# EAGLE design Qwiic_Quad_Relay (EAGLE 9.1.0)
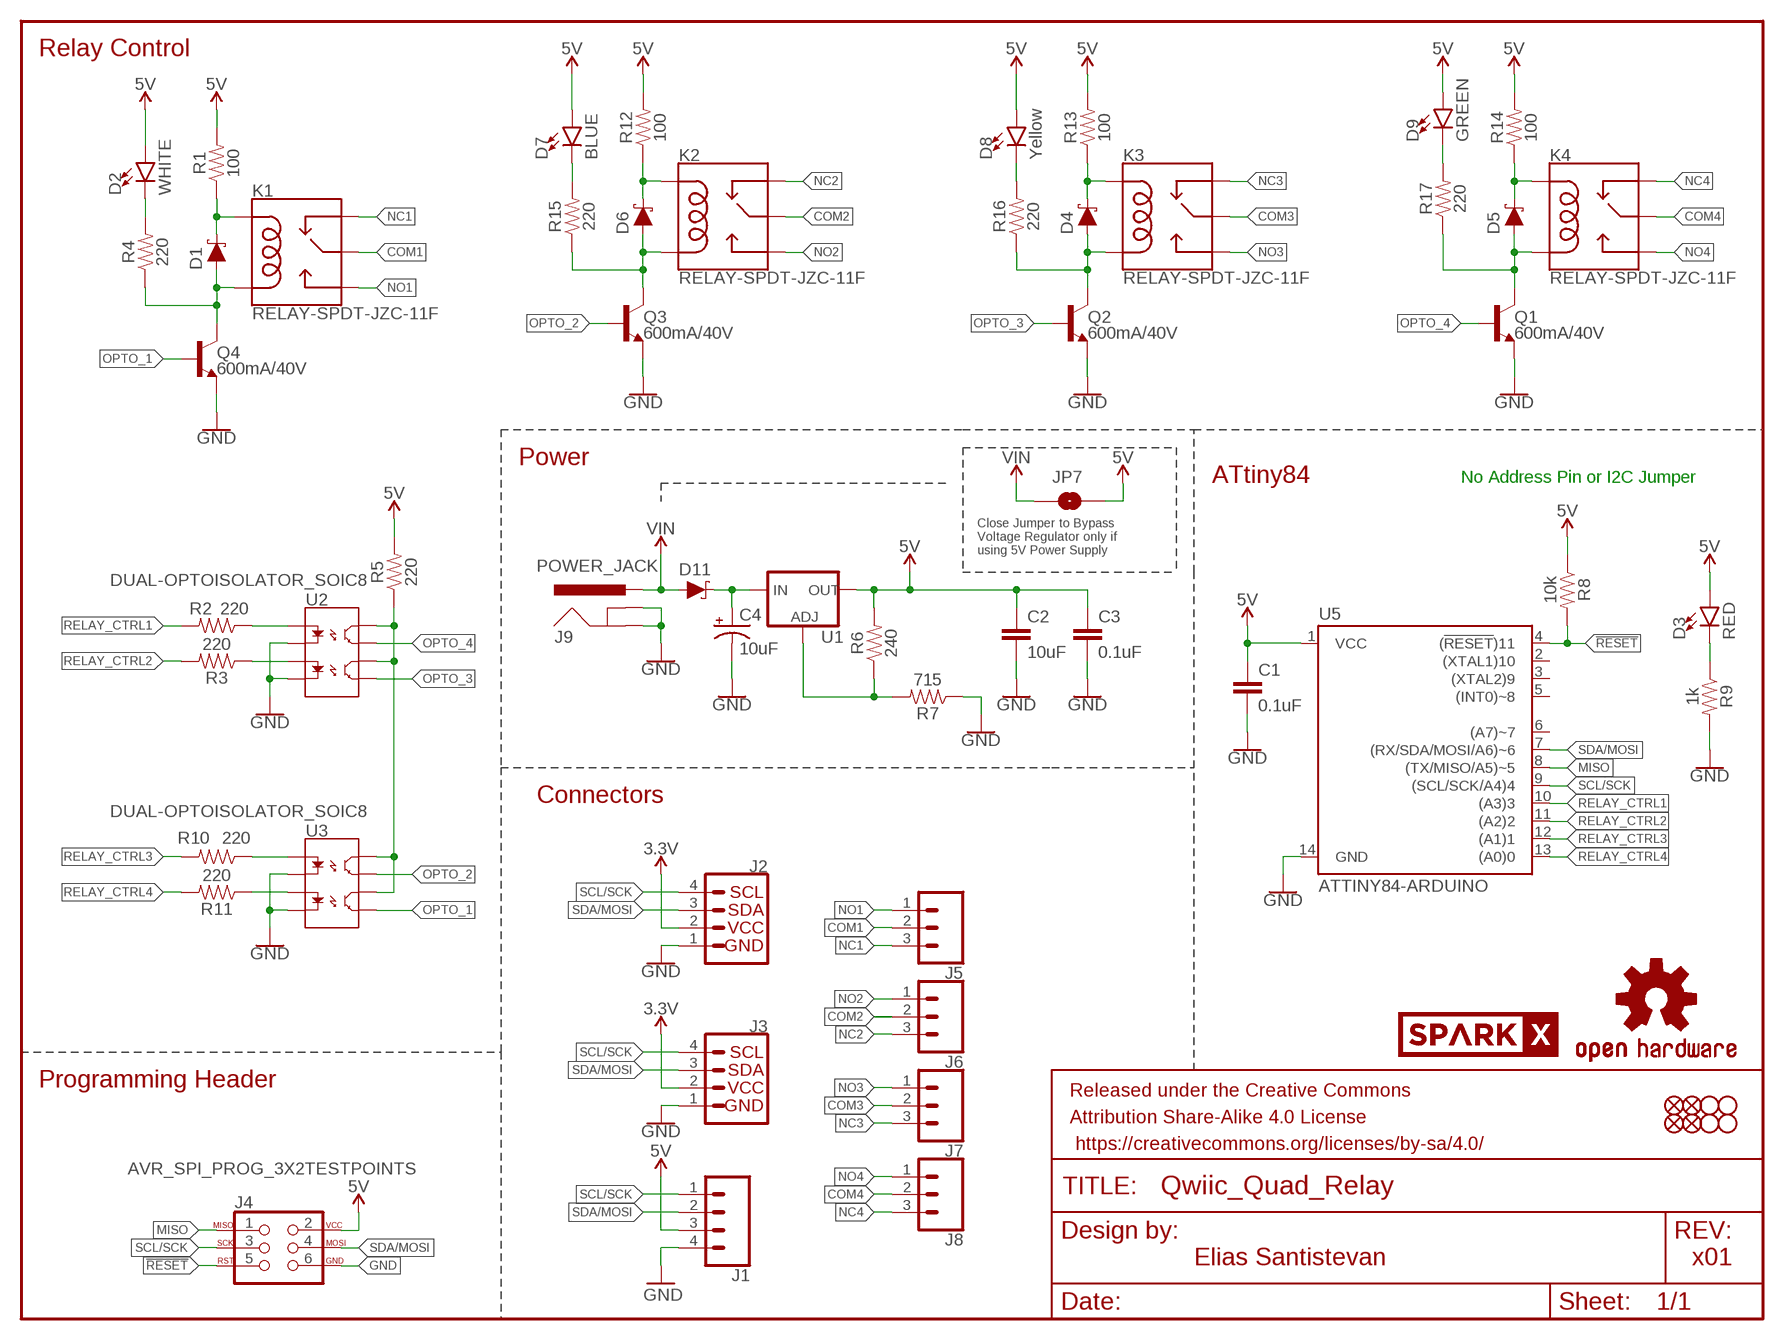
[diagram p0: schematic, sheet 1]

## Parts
C1  0.1uF  0.1UF-0603-25V-(+80/-20%)  [0603]
C2  10uF  10UF-0603-6.3V-20%  [0603]
C3  0.1uF  0.1UF-0603-25V-(+80/-20%)  [0603]
C4  10uF  10UF-POLAR-EIA3528-20V-10%(TANT)  [EIA3528]
D1  1A/23V/620mV  DIODE-SCHOTTKY-BAT20J  [SOD-323]
D2  WHITE  LED-WHITE0603  [LED-0603]
D3  RED  LED-RED0603  [LED-0603]
D4  1A/23V/620mV  DIODE-SCHOTTKY-BAT20J  [SOD-323]
D5  1A/23V/620mV  DIODE-SCHOTTKY-BAT20J  [SOD-323]
D6  1A/23V/620mV  DIODE-SCHOTTKY-BAT20J  [SOD-323]
D7  BLUE  LED-BLUE0603  [LED-0603]
D8  Yellow  LED-YELLOW0603  [LED-0603]
D9  GREEN  LED-GREEN0603  [LED-0603]
D11  1A/40V/500mV  DIODE-SCHOTTKY-SS14  [SMA-DIODE]
FRAME1  FRAME-LETTER  [CREATIVE_COMMONS]
J1  CONN_041X04_NO_SILK  [1X04_NO_SILK]
J2  Qwiic Right Angle  I2C_STANDARDQWIIC  [1X04_1MM_RA]
J3  Qwiic Right Angle  I2C_STANDARDQWIIC  [1X04_1MM_RA]
J4  AVR_SPI_PROG_3X2TESTPOINTS  [2X3_TEST_POINTS]
J5  CONN_03-SCREW-5MM  [SCREWTERMINAL-5MM-3]
J6  CONN_03-SCREW-5MM  [SCREWTERMINAL-5MM-3]
J7  CONN_03-SCREW-5MM  [SCREWTERMINAL-5MM-3]
J8  CONN_03-SCREW-5MM  [SCREWTERMINAL-5MM-3]
J9  POWER_JACK  [POWER_JACK_PTH]
JP1  STAND-OFF  [STAND-OFF]
JP2  FIDUCIAL1X2  [FIDUCIAL-1X2]
JP3  STAND-OFF  [STAND-OFF]
JP4  STAND-OFF  [STAND-OFF]
JP5  STAND-OFF  [STAND-OFF]
JP6  FIDUCIAL1X2  [FIDUCIAL-1X2]
JP7  JUMPER-SMT_2_NO_SILK  [SMT-JUMPER_2_NO_SILK]
JP8  FIDUCIAL1X2  [FIDUCIAL-1X2]
JP9  FIDUCIAL1X2  [FIDUCIAL-1X2]
K1  RELAY-SPDT-JZC-11F  [RELAY-JZC]
K2  RELAY-SPDT-JZC-11F  [RELAY-JZC]
K3  RELAY-SPDT-JZC-11F  [RELAY-JZC]
K4  RELAY-SPDT-JZC-11F  [RELAY-JZC]
LOGO1  OSHW-LOGOS  [OSHW-LOGO-S]
Q1  600mA/40V  TRANS_NPN-MMBT2222AL  [SOT23-3]
Q2  600mA/40V  TRANS_NPN-MMBT2222AL  [SOT23-3]
Q3  600mA/40V  TRANS_NPN-MMBT2222AL  [SOT23-3]
Q4  600mA/40V  TRANS_NPN-MMBT2222AL  [SOT23-3]
R1  100  100OHM-0603-1/10W-1%  [0603]
R2  220  220OHM-0603-1/10W-1%  [0603]
R3  220  220OHM-0603-1/10W-1%  [0603]
R4  220  220OHM-0603-1/10W-1%  [0603]
R5  220  220OHM-0603-1/10W-1%  [0603]
R6  240  240OHM-0603-1/10W-1%  [0603]
R7  715  715OHM-0603-1/10W-1%  [0603]
R8  10k  10KOHM-0603-1/10W-1%  [0603]
R9  1k  1KOHM-0603-1/10W-1%  [0603]
R10  220  220OHM-0603-1/10W-1%  [0603]
R11  220  220OHM-0603-1/10W-1%  [0603]
R12  100  100OHM-0603-1/10W-1%  [0603]
R13  100  100OHM-0603-1/10W-1%  [0603]
R14  100  100OHM-0603-1/10W-1%  [0603]
R15  220  220OHM-0603-1/10W-1%  [0603]
R16  220  220OHM-0603-1/10W-1%  [0603]
R17  220  220OHM-0603-1/10W-1%  [0603]
U1  V_REG_LM1117SOT223  [SOT223]
U2  DUAL-OPTOISOLATOR_SOIC8  [SO08]
U3  DUAL-OPTOISOLATOR_SOIC8  [SO08]
U5  ATTINY84-ARDUINO  [SO14]
U$12  SPARKX-LOGO4  [SPARKX-MEDIUM]

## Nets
3.3V: J2.2 J3.2
5V: C1.1 C2.1 C3.1 D2.A D3.A D7.A D8.A D9.A J1.3 J4.2 JP7.2 R1.2 R5.2 R6.2 R8.1 R12.2 R13.2 R14.2 U1.2(OUT) U1.4(OUT) U5.1(VCC)
!RESET: J4.5 R8.2 U5.4((!RESET!)11)
COM1: J5.2 K1.4(MAIN)
COM2: J6.2 K2.4(MAIN)
COM3: J7.2 K3.4(MAIN)
COM4: J8.2 K4.4(MAIN)
GND: C1.2 C2.2 C3.2 C4.C(-) J1.4 J2.1 J3.1 J4.6 J9.GND J9.GNDBREAK Q1.2(E) Q2.2(E) Q3.2(E) Q4.2(E) R7.1 R9.2 U2.2(C1) U2.4(C2) U3.2(C1) U3.4(C2) U5.14(GND)
MISO: J4.1 U5.8((TX/MISO/A5)~5)
N$1: D6.C K2.5(COIL1) R12.1
N$2: D1.A K1.1(COIL2) Q4.3(C) R4.1
N$3: R11.1 U3.3(A2)
N$4: C4.A(+) D11.C U1.3(IN)
N$5: R10.1 U3.1(A1)
N$6: R5.1 U2.6(CL2) U2.8(CL1) U3.6(CL2) U3.8(CL1)
N$7: D1.C K1.5(COIL1) R1.1
N$8: D2.C R4.2
N$9: R2.1 U2.1(A1)
N$11: R3.1 U2.3(A2)
N$12: D6.A K2.1(COIL2) Q3.3(C) R15.1
N$13: D3.C R9.1
N$14: D4.C K3.5(COIL1) R13.1
N$15: D4.A K3.1(COIL2) Q2.3(C) R16.1
N$16: D5.C K4.5(COIL1) R14.1
N$17: D5.A K4.1(COIL2) Q1.3(C) R17.1
N$19: R6.1 R7.2 U1.1(ADJ)
N$20: D9.C R17.2
N$21: D8.C R16.2
N$22: D7.C R15.2
NC1: J5.3 K1.2(NC)
NC2: J6.3 K2.2(NC)
NC3: J7.3 K3.2(NC)
NC4: J8.3 K4.2(NC)
NO1: J5.1 K1.3(NO)
NO2: J6.1 K2.3(NO)
NO3: J7.1 K3.3(NO)
NO4: J8.1 K4.3(NO)
OPTO_1: Q4.1(B) U3.5(EM2)
OPTO_2: Q3.1(B) U3.7(EM1)
OPTO_3: Q2.1(B) U2.5(EM2)
OPTO_4: Q1.1(B) U2.7(EM1)
RELAY_CTRL1: R2.2 U5.10((A3)3)
RELAY_CTRL2: R3.2 U5.11((A2)2)
RELAY_CTRL3: R10.2 U5.12((A1)1)
RELAY_CTRL4: R11.2 U5.13((A0)0)
SCL/SCK: J1.1 J2.4 J3.4 J4.3 U5.9((SCL/SCK/A4)4)
SDA/MOSI: J1.2 J2.3 J3.3 J4.4 U5.7((RX/SDA/MOSI/A6)~6)
VIN: D11.A J9.PWR JP7.1
Unconnected: U5.2((XTAL1)10) U5.3((XTAL2)9) U5.5((INT0)~8) U5.6((A7)~7)

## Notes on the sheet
- Relay Control
- Power
- ATtiny84 | No Address Pin or I2C Jumper
- Close Jumper to Bypass
  Voltage Regulator only if 
  using 5V Power Supply
- Connectors
- Programming Header
- Elias Santistevan | x01

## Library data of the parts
C1 C3 = SparkFun-Capacitors:0.1UF: 0.1µF ceramic capacitors; PROD_ID: CAP-00810
C2 = SparkFun-Capacitors:10UF: 10.0µF ceramic capacitors; PROD_ID: CAP-11015
C4 = SparkFun-Capacitors:10UF-POLAR: 10.0µF polarized capacitors; PROD_ID: CAP-08063
D1 D4-D6 = SparkFun-DiscreteSemi:DIODE-SCHOTTKY: Schottky diode; PROD_ID: DIO-11623
D2 = SparkFun-LED:LED-WHITE: White SMD LED; PROD_ID: DIO-09004
D3 = SparkFun-LED:LED-RED: Red SMD LED; PROD_ID: DIO-00819
D7 = SparkFun-LED:LED-BLUE: Blue SMD LED; PROD_ID: DIO-08575
D8 = SparkFun-LED:LED-YELLOW: Yellow SMD LED; PROD_ID: DIO-09003
D9 = SparkFun-LED:LED-GREEN: Green SMD LED; PROD_ID: DIO-00821
D11 = SparkFun-DiscreteSemi:DIODE-SCHOTTKY: Schottky diode; PROD_ID: DIO-08053
FRAME1 = SparkFun-Aesthetics:FRAME-LETTER: Schematic Frame - Letter
J1 = SparkFun-Connectors:CONN_04: Multi connection point. Often used as Generic Header-pin footprint for 0.1 inch spaced/style header connections On any of the 0.1 inch spaced packages, you can populate with these: Break Away Headers - Straight (PRT-00116) Break Away Male Headers - Right Angle (PRT-00553) Female Headers (PRT-00115)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; PROD_ID: CONN-09696
J2 J3 = SparkFun-Connectors:I2C_STANDARD: SparkFun I2C Standard Pinout Header SparkFun has standardized on a pinout for all I2C based sensor breakouts. This pinout allows I2C boards to be plugged directly into the headers on Arduino Uno compatible boards, and to be daisy chained easily. Example SparkFun Products: SparkFun Atmospheric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; PROD_ID: CONN-13694
J4 = SparkFun-Connectors:AVR_SPI_PROG_3X2: AVR ISP 6 Pin This is the reduced ISP connector for AVR programming. Common on Arduino. This footprint will take up less PCB space and can be used with a 10-pin to 6-pin adapter such as SKU: BOB-08508 **Special note about "TEST_POINT" package. The stop mask is on the top side, so if you want your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
J5-J8 = SparkFun-Connectors:CONN_03: Multi connection point. Often used as Generic Header-pin footprint for 0.1 inch spaced/style header connections On any of the 0.1 inch spaced packages, you can populate with these: Break Away Headers - Straight (PRT-00116) Break Away Male Headers - Right Angle (PRT-00553) Female Headers (PRT-00115)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; PROD_ID: CONN-10134; SF_SKU: PRT-08433
J9 = SparkFun-Connectors:POWER_JACK: Power Jack Connector This is the standard 5.5mm barrel jack for power. The PTH is the most common, proven, reliable, footprint. The Slot footprint only works if the mill layer is transmitted to the PCB fab house so be warned. Here are the connectors we sell at SparkFun: DC Barrel Power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; PROD_ID: CONN-08197
JP1 JP3-JP5 = SparkFun:STAND-OFF: Stand Off
JP2 JP6 JP8 JP9 = SparkFun-Aesthetics:FIDUCIAL: Fiducial Alignment Points
JP7 = SparkFun-Jumpers:JUMPER-SMT_2_NO: Normally open jumper
K1-K4 = SparkFun-Electromechanical:RELAY-SPDT: SPDT Electromechanical Relay Single-pole, double-throw sealed relays. When current is applied to the coil, it throws a simple changeover switch, terminating the connection from the NC contact to ground and closing the NO contact. Use them to switch high voltage/high current devices. SparkFun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; PROD_ID: COMP-09533; SF_SKU: COM-00100
LOGO1 = SparkFun-Aesthetics:OSHW-LOGO: Open-Source Hardware (OSHW) Logo
Q1-Q4 = SparkFun-DiscreteSemi:TRANS_NPN: NPN transistor Current controlled devices typically used to amplify current or used as a switch. BC547 - COM-08928 (TO-92 45V 100mA) (1.Collector 2.Base 3.Emitter) 2N3904 - COM-00521 (TO-92 40V 200mA) (1.Emitter 2.Base 3.Collector) P2N2222A - COM-12852 (TO-92 40V 600mA) (1.Collector 2.Base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; PROD_ID: TRANS-08049
R1 R12-R14 = SparkFun-Resistors:100OHM: 100Ω resistor; PROD_ID: RES-07863
R2-R5 R10 R11 R15-R17 = SparkFun-Resistors:220OHM: 220Ω resistor; PROD_ID: RES-07861
R6 = SparkFun-Resistors:240OHM: 240Ω resistor; PROD_ID: RES-07849
R7 = SparkFun-Resistors:715OHM: 715Ω resistor; PROD_ID: RES-07850
R8 = SparkFun-Resistors:10KOHM: 10kΩ resistor; PROD_ID: RES-00824
R9 = SparkFun-Resistors:1KOHM: 1kΩ resistor; PROD_ID: RES-07856
U1 = SparkFun-IC-Power:V_REG_LM1117: Voltage Regulator LM1117 Standard adjustable voltage regulator but in SMD form. Spark Fun Electronics SKU : COM-00595; PROD_ID: VREG-08170
U2 U3 = SparkFun-DiscreteSemi:DUAL-OPTOISOLATOR: Optocoupler, Phototransistor Output, Dual Channel Optically coupled pairs with a gallium arsenide infrared LED and a silicon NPN phototransistor. Signal information, including a DC level, can be transmitted by the device while maintaining a high degree of electrical isolation between input and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; PROD_ID: IC-09076
U5 = SparkFun-IC-Microcontroller:ATTINY84-ARDUINO; PROD_ID: IC-11285
U$12 = SparkX:SPARKX-LOGO

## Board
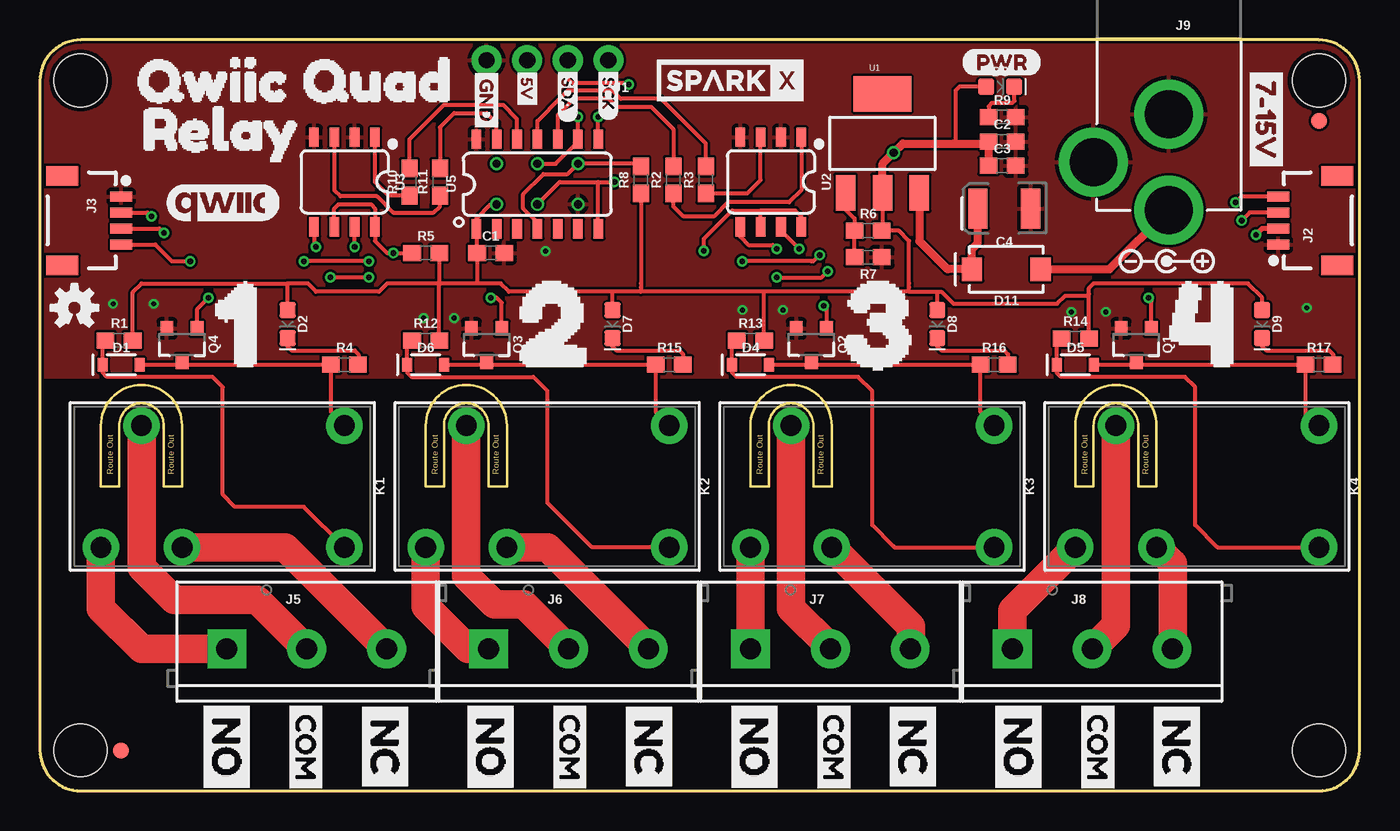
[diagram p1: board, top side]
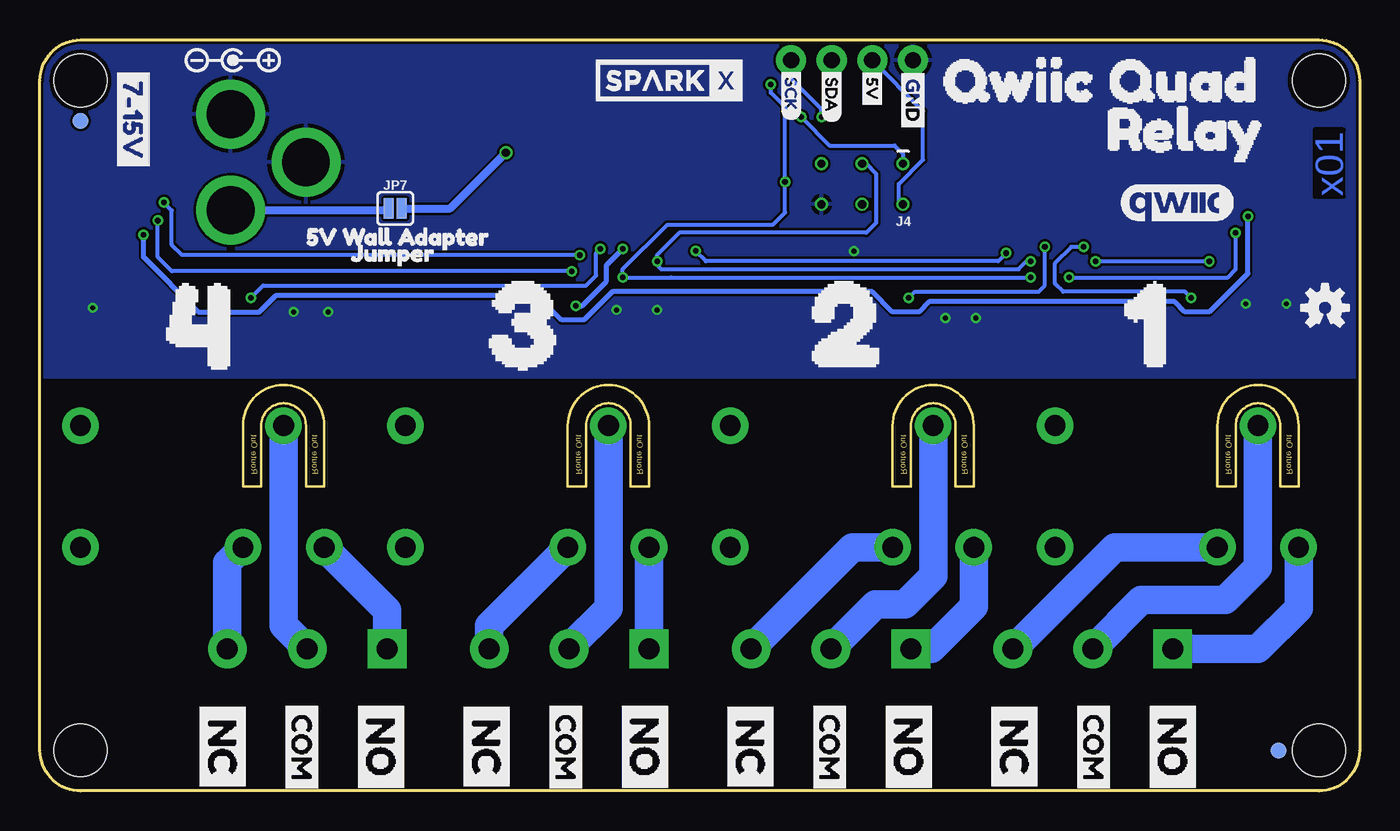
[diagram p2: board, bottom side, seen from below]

Size 82.55 x 46.99 mm. Coordinates in mm from the lower left corner, seen from the top.
Outline: 80.01,46.99 2.54,46.99 arc90 0,44.45 0,2.54 arc90 2.54,0 80.01,0 arc90 82.55,2.54 82.55,44.45 arc90 80.01,46.99
Copper layers (1*16): Top 0.035mm / dielectric 1.5mm / Bottom 0.035mm
Design rules "SparkFun-2-layer-PCBWay-LIMIT": minimum track width 6mil, minimum drill 0.3mm, track to track 6mil, track to pad 6mil, pad to pad 6mil, via to via 6mil, smd to smd 6mil, copper to edge 6mil, drill to drill 6mil, minimum pad ring 6mil, minimum via ring 6mil, stop-mask expansion 4mil, vias tented up to drill 25mil, thermal gap 10mil
Milling: 40 lines

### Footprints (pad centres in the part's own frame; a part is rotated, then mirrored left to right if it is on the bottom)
0603 = smd 1.1 x 1: 1 -0.85,0; 2 0.85,0
EIA3528 = smd 1.2 x 2.5: A 1.65,0; C -1.65,0
SOD-323 = smd 0.63 x 0.83: A 1.15,0; C -1.15,0
LED-0603 = smd 1 x 1: A -0.877,0; C 0.877,0
SMA-DIODE = smd 1.27 x 1.47: A -2.15,0; C 2.15,0
1X04_NO_SILK = drill 1.016 pad 1.88: 1 0,0; 2 2.54,0; 3 5.08,0; 4 7.62,0
1X04_1MM_RA = smd 0.6 x 1.35: 1 -1.5,0; 2 -0.5,0; 3 0.5,0; 4 1.5,0 | smd 1.2 x 2: NC1 2.8,-3.675; NC2 -2.8,-3.675
2X3_TEST_POINTS = drill 0.508: 1 -2.54,-1.27; 2 -2.54,1.27; 3 0,-1.27; 4 0,1.27; 5 2.54,-1.27; 6 2.54,1.27
SCREWTERMINAL-5MM-3 = drill 1.3 pad 2.413 square: 1 0,0 | drill 1.3 pad 2.413: 2 5,0; 3 10,0
POWER_JACK_PTH = drill 2.997 pad 4.318: GND 0,7.7; GNDBREAK 4.7,10.7; PWR 0,13.7
STAND-OFF = hole 3.302: 0,0
FIDUCIAL-1X2 = smd 1 x 1: 1 0,0
SMT-JUMPER_2_NO_SILK = smd 0.635 x 1.27: 1 -0.406,0; 2 0.406,0
RELAY-JZC = drill 1.3 pad 2.286: 1 3.81,-8.89; 2 -3.81,1.27; 3 -3.81,6.35; 4 3.81,3.81; 5 -3.81,-8.89
SOT23-3 = smd 0.8 x 0.9: 1 -0.95,-1; 2 0.95,-1; 3 0,1.1
SOT223 = smd 1.219 x 2.235: 1 -2.311,-3.099; 2 0,-3.099; 3 2.311,-3.099 | smd 3.6 x 2.2: 4 0,3.099
SO08 = smd 0.6 x 1.2: 1 -1.905,-2.8; 2 -0.635,-2.8; 3 0.635,-2.8; 4 1.905,-2.8; 5 1.905,2.8; 6 0.635,2.8; 7 -0.635,2.8; 8 -1.905,2.8
SO14 = smd 0.6 x 1.2: 1 -3.175,-2.8; 2 -1.905,-2.8; 3 -0.635,-2.8; 4 0.635,-2.8; 5 1.905,-2.8; 6 3.175,-2.8; 7 4.445,-2.8; 8 4.445,2.8; 9 3.175,2.8; 10 1.905,2.8; 11 0.635,2.8; 12 -0.635,2.8; 13 -1.905,2.8; 14 -3.175,2.8

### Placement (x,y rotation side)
C1  28.19,33.66 0 top
C2  60.2,40.64 0 top
C3  60.2,39.12 0 top
C4  60.33,36.45 180 top
D1  5.08,26.67 0 top
D2  15.49,29.21 270 top
D3  60.07,44.07 0 top
D4  44.45,26.67 0 top
D5  64.77,26.67 0 top
D6  24.13,26.67 0 top
D7  35.81,29.21 270 top
D8  56.13,29.21 270 top
D9  76.45,29.21 270 top
D11  60.45,32.64 180 top
FRAME1  not placed on the board
J1  35.56,45.72 180 top
J2  77.47,35.69 90 top
J3  5.08,35.69 270 top
J4  31.11,37.97 180 bottom
J5  11.68,8.89 0 top
J6  28.07,8.89 0 top
J7  44.45,8.89 0 top
J8  60.83,8.89 0 top
J9  70.61,50.04 180 top
JP1  2.54,2.54 0 top
JP2  80.01,41.91 0 bottom
JP3  2.54,44.45 0 top
JP4  80.01,44.45 0 top
JP5  80.01,2.54 0 top
JP6  5.08,2.54 0 bottom
JP7  60.33,36.45 0 bottom
JP8  5.08,2.54 0 top
JP9  80.01,41.91 0 top
K1  10.16,19.05 90 top
K2  30.48,19.05 90 top
K3  50.8,19.05 90 top
K4  71.12,19.05 90 top
LOGO1  2.16,30.23 0 top
Q1  68.58,27.94 180 top
Q2  48.26,27.94 180 top
Q3  27.94,27.94 180 top
Q4  8.89,27.94 180 top
R1  4.95,28.19 0 top
R2  39.62,38.23 90 top
R3  41.66,38.23 90 top
R4  19.05,26.67 0 top
R5  24.13,33.66 0 top
R6  51.82,35.05 0 top
R7  51.82,33.4 180 top
R8  37.59,38.23 90 top
R9  60.2,42.16 0 top
R10  23.11,38.1 90 top
R11  25.02,38.1 90 top
R12  24.13,28.19 0 top
R13  44.45,28.19 0 top
R14  64.77,28.32 0 top
R15  39.37,26.67 0 top
R16  59.69,26.67 0 top
R17  80.01,26.67 0 top
U1  52.7,40.51 0 top
U2  45.72,38.1 180 top
U3  19.05,38.1 180 top
U5  30.48,37.97 0 top
U$1  [PWR-()-04]  57.66,45.59 0 top
U$2  [20]  25.4,29.21 0 top
U$3  [10]  6.35,29.21 0 top
U$4  [30]  45.72,29.21 0 top
U$5  [40]  66.04,29.21 0 top
U$6  [QWIIC_QUAD_0]  3.81,44.45 0 top
U$7  [RELAY0]  4.19,41.4 0 top
U$8  [SCK-[)-03]  35.56,45.34 270 top
U$9  [GND-03]  27.94,45.34 270 top
U$10  [5V0]  30.48,45.34 270 top
U$11  [SDA0]  33.02,45.34 270 top
U$12  43.18,44.45 0 top
U$13  [OSHW-LOGO-S]  2.16,30.23 0 bottom
U$14  [SPARKX-MEDIUM]  43.18,44.45 0 bottom
U$15  [NO0]  11.68,6.22 270 top
U$16  [COM0]  16.64,5.97 270 top
U$17  [NC0]  21.59,6.1 270 top
U$18  [NO0]  28.19,6.22 270 top
U$19  [COM0]  33.15,5.97 270 top
U$20  [NC0]  38.1,6.1 270 top
U$21  [NO0]  44.7,6.22 270 top
U$22  [COM0]  49.66,5.97 270 top
U$23  [NC0]  54.61,6.1 270 top
U$24  [NO0]  61.21,6.22 270 top
U$25  [COM0]  66.17,5.97 270 top
U$26  [NC0]  71.12,6.1 270 top
U$27  [NO0]  44.7,6.22 270 bottom
U$28  [COM0]  66.17,5.97 270 bottom
U$29  [NC0]  71.12,6.1 270 bottom
U$30  [NO0]  61.21,6.22 270 bottom
U$31  [COM0]  49.66,5.97 270 bottom
U$32  [NC0]  54.61,6.1 270 bottom
U$33  [NO0]  28.19,6.22 270 bottom
U$34  [COM0]  33.15,5.97 270 bottom
U$35  [NC0]  38.1,6.1 270 bottom
U$36  [NO0]  11.68,6.22 270 bottom
U$37  [COM0]  16.64,5.97 270 bottom
U$38  [NC0]  21.59,6.1 270 bottom
U$39  [10]  19.3,29.21 0 bottom
U$40  [20]  38.86,29.21 0 bottom
U$41  [30]  59.05,29.21 0 bottom
U$42  [40]  79.25,29.08 0 bottom
U$43  [QWIIC_QUAD_0]  28.32,44.45 0 bottom
U$44  [RELAY0]  18.03,41.4 0 bottom
U$45  [GND-03]  27.94,45.34 270 bottom
U$46  [5V0]  30.48,45.34 270 bottom
U$47  [SDA0]  33.02,45.34 270 bottom
U$48  [SCK-[)-03]  35.56,45.34 270 bottom
U$49  [7#15V0]  76.71,45.59 270 top
U$50  [5V_WALL_ADAPTER0]  66.8,34.67 0 bottom
U$51  [POLARITY_MARKING_CENTER_POSITIVE#JPG]  70.48,33.15 0 top
U$52  [JUMPER0]  64.01,33.66 0 bottom
U$53  [7#15V0]  76.71,45.59 270 bottom
U$54  [POLARITY_MARKING_CENTER_POSITIVE#JPG]  70.48,45.72 0 bottom
U$55  [QWIIC#JPG]  11.43,36.83 0 top
U$57  [QWIIC#JPG]  11.43,36.83 0 bottom

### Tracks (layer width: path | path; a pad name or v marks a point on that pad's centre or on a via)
3.3V  (via drill 0.35)
  Top 0.254: J3.2 6.74,36.19 v6.99,35.94
  Top 0.305: J2.2 76.46,35.19 v76.07,34.8
  Bottom 0.305: v6.99,35.94 6.99,32.38 9.4,29.97 10.92,29.97 11.56,30.61 26.92,30.61 27.56,29.97 29.21,29.97 30.48,31.24 46.74,31.24 48.51,29.46 49.91,29.46 51.44,30.99 67.82,30.99 68.83,29.97 72.64,29.97 76.07,33.4 v76.07,34.8
5V  (via drill 0.51)
  Top 0.254: 54.37,31.24 45.3,31.24 | 45.3,31.24 37.59,31.24 | R8.1 37.59,31.75 37.59,31.5 37.59,31.24 | 15.49,31.75 6.35,31.75 5.8,31.2 R1.2 | D9.A 76.45,30.86 75.56,31.75 65.91,31.75 65.66,31.5 65.62,31.46 65.62,31.11 | D2.A 15.49,31.75 | J4.2 28.19,36.7 27.3,35.81 U5.1 27.34,35.13 C1.1 27.34,31.79 27.3,31.75 | D3.A 57.53,44.07 57.28,43.81 57.28,40.64 57.15,40.51 | U1.2 52.7,35.09 | 52.7,35.09 R6.2 | 52.7,35.09 52.74,35.05 53.72,35.05 54.37,34.41 54.37,31.75 54.37,31.5 54.37,31.24 | R14.2 65.62,31.11 | R13.2 45.3,31.24 | 37.59,31.24 35.81,31.24 | 35.81,31.24 29.34,31.24 28.83,31.75 27.3,31.75 | 27.3,31.75 25.02,31.75 | 25.02,31.75 24.89,31.75 | 24.89,31.75 21.72,31.75 21.21,31.24 17.27,31.24 16.76,31.75 15.49,31.75 | R12.2 24.98,31.66 24.89,31.75 | 25.02,31.75 24.98,31.79 R5.2 | D7.A 35.81,31.24 | 54.37,31.24 56.13,31.24 | 56.13,31.24 56.39,31.24 57.15,30.48 63.63,30.48 64.14,30.99 65.49,30.99 65.62,31.11 | D8.A 56.13,31.24
  Top 0.508: C3.1 C2.1 59.22,40.51 57.15,40.51 53.98,40.51 v53.4,39.94 52.7,39.24 U1.2
  Bottom 0.254: J1.3 27.3,42.55 27.3,39.5 28.83,37.97 28.83,36.96 J4.2
  Bottom 0.508: JP7.2 56.9,36.45 v53.4,39.94
!RESET
  Top 0.254: U5.4 31.11,35.55 30.23,36.44 30.23,37.34 31.5,38.61 33.02,38.61 J4.5 37.43,39.24 R8.2
COM1
  Top 1.778: K1.4 6.35,13.97 8.38,11.94 8.89,11.94 13.59,11.94 16.64,8.89 J5.2
  Bottom 1.778: K1.4 6.35,13.97 8.38,11.94 13.64,11.94 J5.2
COM2
  Top 1.778: K2.4 26.67,13.46 28.45,11.68 30.27,11.68 J6.2
  Bottom 1.778: K2.4 26.67,13.46 28.45,11.68 30.27,11.68 J6.2 | J6.2
COM3
  Top 1.778: K3.4 46.99,11.43 49.45,8.97 J7.2
  Bottom 1.778: K3.4 46.99,11.43 49.45,8.97 J7.2
COM4
  Top 1.778: K4.4 67.31,10.37 J8.2 | K4.4
  Bottom 1.778: K4.4 67.31,10.37 J8.2 | K4.4
GND  (via drill 0.3)
  other vias: 46.48,30.1 66.67,29.97 25.91,29.59 7.11,30.48 64.52,29.97 79.25,30.23 43.94,30.1 4.57,30.48 24,29.59 31.62,33.78
  pour Bottom: 0,25.91 82.55,25.91 82.55,46.99 0,46.99
  pour Top: 0,25.91 0,46.99 82.55,46.99 82.55,25.91
MISO  (via drill 0.35)
  Top 0.254: U5.8 v34.92,42.16
  Bottom 0.254: v34.92,42.16 33.15,40.39 29.08,40.39 28.57,39.88 J4.1
N$1
  Top 0.254: K2.5 34.54,15.24 31.75,18.03 31.75,25.02 30.99,25.78 30.86,25.91 23.24,25.91 22.98,26.17 D6.C 22.98,27.89 R12.1
N$2
  Top 0.254: D1.A 8.72,26.67 Q4.3 9.06,26.67 R4.1 18.2,23.71 K1.1
N$3
  Top 0.254: U3.3 18.41,37.59 18.8,37.21 21.08,37.21 22.1,36.2 24.64,36.2 25.02,36.58 R11.1
N$4
  Top 0.508: U1.3 55.02,34.39 56.13,33.27 56.77,32.64 D11.C 58.3,33.92 58.67,34.29 C4.A
N$5
  Top 0.254: R10.1 21.8,37.25 20.95,38.1 U3.1
N$6  (via drill 0.35)
  Top 0.254: U3.6 18.41,36.45 18.67,36.7 20.7,36.7 20.95,36.45 U3.8 20.95,34.42 21.72,33.66 v22.1,33.66 R5.1 | 45.09,36.32 46.99,36.32 47.24,36.32 47.62,35.94 U2.8 | U2.6 45.09,36.32 | v41.53,33.78 41.53,34.54 43.31,36.32 45.09,36.32
  Bottom 0.254: v41.53,33.78 40.89,33.15 22.61,33.15 v22.1,33.66
N$7
  Top 0.254: R1.1 3.93,28.02 D1.C 3.93,26.17 4.19,25.91 10.79,25.91 11.43,25.27 11.43,18.54 12.19,17.78 16.51,17.78 K1.5
N$8
  Top 0.254: R4.2 19.93,26.7 19.93,27.32 19.68,27.56 15.75,27.56 15.49,27.81 D2.C
N$9
  Top 0.254: U2.1 47.62,37.59 46.86,36.83 43.05,36.83 42.16,35.94 40.26,35.94 39.62,36.58 R2.1
N$11
  Top 0.254: U2.3 45.09,38.23 44.23,37.38 R3.1
N$12
  Top 0.254: K2.1 38.52,23.71 R15.1 28.11,26.67 Q3.3 27.77,26.67 D6.A
N$13
  Top 0.254: D3.C 60.96,44.06 60.96,43.18 60.83,43.05 59.56,43.05 59.35,42.84 R9.1
N$14
  Top 0.254: R13.1 43.3,27.89 D4.C 43.3,26.17 43.56,25.91 51.18,25.91 52.07,25.02 | 52.07,25.02 52.07,16.64 53.4,15.3 53.47,15.24 K3.5 | 52.07,25.02 arc90 52.07,25.02
N$15
  Top 0.254: D4.A 48.09,26.67 Q2.3 48.43,26.67 R16.1 58.84,23.71 K3.1
N$16
  Top 0.254: 72.26,16.64 73.66,15.24 K4.5 | R14.1 63.62,28.02 D5.C 63.63,26.16 63.88,25.91 71.63,25.91 72.26,25.27 72.26,16.64 | 72.26,16.64
N$17
  Top 0.254: D5.A 68.41,26.67 Q1.3 68.75,26.67 R17.1 79.16,22.86 K4.1
N$19
  Top 0.254: U1.1 50.39,36.39 50.97,35.81 R6.1 R7.2
N$20
  Top 0.254: R17.2 80.89,26.7 80.9,26.71 80.9,27.3 80.64,27.56 76.71,27.56 76.45,27.81 D9.C
N$21
  Top 0.254: R16.2 60.57,26.7 60.57,27.32 60.33,27.56 56.39,27.56 56.13,27.81 D8.C
N$22
  Top 0.254: D7.C 35.81,27.81 36.07,27.56 40.01,27.56 40.22,27.34 R15.2
NC1
  Top 1.778: K1.2 15.33,15.24 J5.3
  Bottom 1.778: K1.2 15.32,15.24 21.67,8.89 J5.3
NC2
  Top 1.778: K2.2 31.75,15.24 38.07,8.92 J6.3
  Bottom 1.778: K2.2 31.72,15.24 J6.3
NC3
  Top 1.778: K3.2 54.48,10.29 54.48,8.92 J7.3
  Bottom 1.778: K3.2 54.45,10.32 J7.3
NC4
  Top 1.778: K4.2 70.87,14.22 70.87,8.92 J8.3
  Bottom 1.778: K4.2 70.83,14.26 J8.3
NO1
  Top 1.778: K1.3 3.81,11.43 6.35,8.89 J5.1
  Bottom 1.778: J5.1 6.35,8.89 3.81,11.43 K1.3
NO2
  Top 1.778: J6.1 26.8,8.89 24.13,11.56 K2.3
  Bottom 1.778: J6.1 26.8,8.89 24.13,11.56 K2.3
NO3
  Top 1.778: J7.1 K3.3
  Bottom 1.778: J7.1 K3.3
NO4
  Top 1.778: J8.1 60.83,11.3 K4.3
  Bottom 1.778: J8.1 60.83,11.3 K4.3
OPTO_1  (via drill 0.35)
  Top 0.254: Q4.1 9.84,30.16 v10.54,30.86 | U3.5 17.14,34.16 v17.27,34.04
  Bottom 0.254: v10.54,30.86 10.92,31.24 18.54,31.24 19.05,31.75 19.05,33.02 18.03,34.04 v17.27,34.04
OPTO_2  (via drill 0.35)
  Top 0.254: v19.68,34.04 U3.7 | v28.19,30.86 28.57,30.86 28.89,30.55 Q3.1
  Bottom 0.254: v19.68,34.04 19.68,31.62 20.07,31.24 27.81,31.24 v28.19,30.86
OPTO_3  (via drill 0.35)
  Top 0.254: U2.5 43.81,34.67 44.32,34.16 45.85,34.16 v46.1,33.91 | Q2.1 49.21,30.16 v49.02,30.35
  Bottom 0.305: v46.1,33.91 47.12,32.89 47.12,31.88 48.64,30.35 v49.02,30.35
OPTO_4  (via drill 0.35)
  Top 0.254: Q1.1 69.53,30.67 v69.34,30.86 | U2.7 46.48,35.3 46.48,34.92 v47.5,33.91
  Bottom 0.254: v69.34,30.86 68.58,31.62 48.39,31.62 47.75,32.26 47.75,33.66 v47.5,33.91
RELAY_CTRL1
  Top 0.254: U5.10 32.38,42.29 33.4,43.31 35.56,43.31 36.07,42.8 38.23,42.8 39.62,41.4 R2.2
RELAY_CTRL2
  Top 0.254: U5.11 | U5.11 31.11,41.91 32.51,43.31 33.02,43.81 35.81,43.81 36.32,43.31 38.86,43.31 41.66,40.51 R3.2
RELAY_CTRL3
  Top 0.254: R10.2 23.11,40.77 25.27,42.93 28.96,42.93 29.84,42.04 U5.12
RELAY_CTRL4
  Top 0.254: U5.13 28.57,41.78 27.94,42.42 25.91,42.42 25.02,41.53 R11.2
SCL/SCK  (via drill 0.35)
  Top 0.254: J2.4 75.16,37.19 v74.8,36.83 | J4.3 32.26,39.24 33.66,40.64 U5.9 v33.66,42.16 | 48.39,33.15 48.26,33.15 | 48.26,33.15 44.2,33.15 v43.94,33.15 | v20.57,33.15 v16.51,33.15 | J3.4 7.21,34.19 8.26,33.15 v9.4,33.15 | 48.26,33.15 48.39,33.15 | 48.39,33.15 v48.77,33.53
  Bottom 0.254: v16.51,33.15 v9.4,33.15 | J1.1 35.56,44.58 33.66,42.67 v33.66,42.16 | J4.3 30.86,39.24 30.23,38.61 30.23,35.56 30.86,34.92 42.55,34.92 43.94,33.53 v43.94,33.15 43.94,32.89 43.69,32.64 21.34,32.64 20.83,33.15 v20.57,33.15 | v74.8,36.83 74.3,36.32 74.3,34.16 73.66,33.53 v48.77,33.53 | v20.57,33.15
SDA/MOSI  (via drill 0.35)
  Top 0.254: v20.57,32.13 v18.16,32.13 | J1.2 33.02,44.58 33.27,44.32 36.7,44.32 v36.83,44.2 | J4.4 32.51,38.1 34.92,38.1 | 34.92,38.1 v35.94,38.1 | U5.7 34.92,38.1 | J3.3 7.49,35.19 v7.75,34.92 | v75.18,35.69 75.68,36.19 J2.3 | v49.28,32.51 48.9,32.13 v46.1,32.13
  Bottom 0.254: v18.16,32.13 8.26,32.13 7.75,32.64 v7.75,34.92 | v35.94,38.1 35.94,36.2 36.7,35.43 43.31,35.43 46.1,32.64 v46.1,32.13 43.05,32.13 v20.57,32.13 | v35.94,38.1 | v35.94,38.1 35.94,42.8 36.83,43.69 v36.83,44.2 | v75.18,35.69 75.18,33.4 74.3,32.51 v49.28,32.51
VIN
  Top 0.508: D11.A 66.91,32.64 J9.PWR
  Bottom 0.508: J9.PWR 60.84,36.34 JP7.1

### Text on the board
Bottom: x01
Milling: Route Out | Route Out | Route Out | Route Out | Route Out | Route Out | Route Out | Route Out
tDocu: Elias Santistevan

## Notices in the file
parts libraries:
SparkFun-PowerSymbols: Licensing: Creative Commons ShareAlike 4.0 International - https://creativecommons.org/licenses/by-sa/4.0
SparkFun-Aesthetics: Released under the Creative Commons Attribution Share-Alike 4.0 License
SparkFun-Aesthetics: https://creativecommons.org/licenses/by-sa/4.0
